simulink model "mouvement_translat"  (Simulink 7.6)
settings: Solver=ode15s  StartTime=0.0  StopTime=5  RelTol=1e-3
StopFcn:
  | close all
  | load pos_vit.mat
  | plot(pv(1,:),pv(2,:))
  | hold on
  | plot(pv(1,:),pv(3,:))
  | 
  | title('Position et vitesse')
  | grid
libraries: fl_lib x8, nesl_utility x5, elec_lib x1

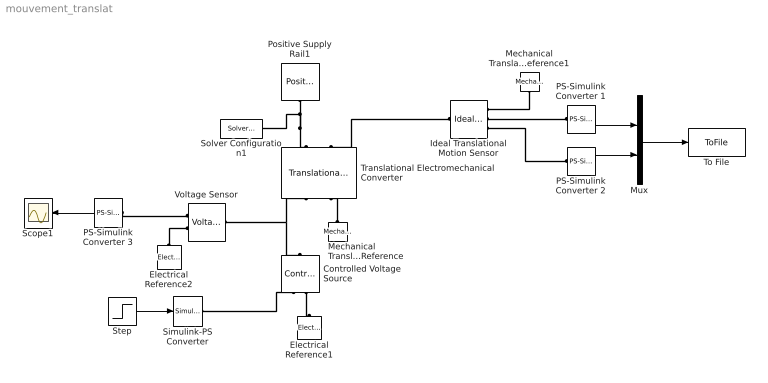
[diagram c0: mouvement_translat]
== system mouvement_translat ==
  Controlled Voltage Source : fl_lib/Electrical/Electrical Sources/Controlled Voltage Source  DialogController=NetworkEngine.DynNeDlgSource  SystemSampleTime=-1  i_Log=off  v_Log=off  LocalVarNames=|i|v  LocalVarDescs=|i|v  LocalVarLogging=[0 0]
  Electrical Reference1 : fl_lib/Electrical/Electrical Elements/Electrical Reference  DialogController=NetworkEngine.DynNeDlgSource  SystemSampleTime=-1  i_Log=off  LocalVarNames=|i  LocalVarDescs=|i  LocalVarLogging=[]
  Electrical Reference2 : fl_lib/Electrical/Electrical Elements/Electrical Reference  DialogController=NetworkEngine.DynNeDlgSource  SystemSampleTime=-1  i_Log=off  LocalVarNames=|i  LocalVarDescs=|i  LocalVarLogging=[]
  Ideal Translational Motion Sensor : fl_lib/Mechanical/Mechanical Sensors/Ideal Translational Motion Sensor  DialogController=NetworkEngine.DynNeDlgSource  SystemSampleTime=-1  offset=0 m  v_Log=off  f_Log=off  x_Log=off  LocalVarNames=|v|f|x  LocalVarDescs=|v|f|x  LocalVarLogging=[0 0 0]
  Mechanical Translational Reference : fl_lib/Mechanical/Translational Elements/Mechanical Translational Reference  DialogController=NetworkEngine.DynNeDlgSource  SystemSampleTime=-1  f_Log=off  LocalVarNames=|f  LocalVarDescs=|f  LocalVarLogging=0
  Mechanical Translational Reference1 : fl_lib/Mechanical/Translational Elements/Mechanical Translational Reference  DialogController=NetworkEngine.DynNeDlgSource  SystemSampleTime=-1  f_Log=off  LocalVarNames=|f  LocalVarDescs=|f  LocalVarLogging=0
  Mux : Mux  Inputs=2
  PS-Simulink Converter 1 : nesl_utility/PS-Simulink Converter  DialogController=NetworkEngine.DynNeUtilDlgSource  SystemSampleTime=-1  PhysicalDomain=network_engine_domain  LeftPortType=input  RightPortType=output  SubClassName=ps_output  Unit=m/s  AffineConversion=off
  PS-Simulink Converter 2 : nesl_utility/PS-Simulink Converter  DialogController=NetworkEngine.DynNeUtilDlgSource  SystemSampleTime=-1  PhysicalDomain=network_engine_domain  LeftPortType=input  RightPortType=output  SubClassName=ps_output  Unit=m  AffineConversion=off
  PS-Simulink Converter 3 : nesl_utility/PS-Simulink Converter  DialogController=NetworkEngine.DynNeUtilDlgSource  SystemSampleTime=-1  PhysicalDomain=network_engine_domain  LeftPortType=input  RightPortType=output  SubClassName=ps_output  Unit=V  AffineConversion=off
  Positive Supply Rail1 : elec_lib/Sources/Positive Supply Rail  DialogController=NetworkEngine.DynNeDlgSource  SystemSampleTime=-1  v0=12 V  current_Log=off  voltage_Log=off  power_Log=off  LocalVarNames=|current|voltage|power  LocalVarDescs=|Current (A)|Voltage (V)|Power (W)  LocalVarLogging=[0 0 0]
  Scope1 : Scope
  Simulink-PS Converter : nesl_utility/Simulink-PS Converter  DialogController=NetworkEngine.DynNeUtilDlgSource  SystemSampleTime=-1  PhysicalDomain=network_engine_domain  LeftPortType=input  RightPortType=output  SubClassName=ps_input  Unit=1  AffineConversion=off  InputFilterTimeConstant=.001  UdotUserProvided=0
  Solver Configuration1 : nesl_utility/Solver Configuration  DialogController=NetworkEngine.DynNeUtilDlgSource  SystemSampleTime=-1  PhysicalDomain=network_engine_domain  LeftPortType=input  RightPortType=generic  SubClassName=solver  Accelerate=off  Profile=off  ResidualTolerance=1e-9  MaxNonlinIter=12  MaxModeIter=2  DoFixedCost=off  UseLocalSampling=off  DoDC=off  LinearAlgebra=Sparse  LocalSolverSampleTime=.001  LocalSolverChoice=NE_BACKWARD_EULER_ADVANCER  UseLocalSolver=off
  Step : Step  Time=0.5  Before=12  After=0  SampleTime=0
  To File : ToFile  Filename=pos_vit.mat  MatrixName=pv
  Translational Electromechanical Converter : fl_lib/Electrical/Electrical Elements/Translational Electromechanical Converter  DialogController=NetworkEngine.DynNeDlgSource  SystemSampleTime=-1  K=0.1 s*V/m  i_Log=off  v_Log=off  f_Log=off  u_Log=off  LocalVarNames=|i|v|f|u  LocalVarDescs=|i|v|f|u  LocalVarLogging=[0 0 0 0]
  Voltage Sensor : fl_lib/Electrical/Electrical Sensors/Voltage Sensor  DialogController=NetworkEngine.DynNeDlgSource  SystemSampleTime=-1  i1_Log=off  v1_Log=off  LocalVarNames=|i1|v1  LocalVarDescs=|i1|v1  LocalVarLogging=[0 0]
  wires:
  PS-Simulink Converter 1/1 -> Mux/1
  PS-Simulink Converter 2/1 -> Mux/2
  Mux/1 -> To File/1
  Step/1 -> Simulink-PS Converter/1
  PS-Simulink Converter 3/1 -> Scope1/1
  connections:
  Voltage Sensor/LConn1 -- Translational Electromechanical Converter/RConn1 -- Controlled Voltage Source/LConn1
  Positive Supply Rail1/RConn1 -- Translational Electromechanical Converter/LConn1 -- Solver Configuration1/RConn1
  Ideal Translational Motion Sensor/LConn1 -- Translational Electromechanical Converter/LConn2
  Mechanical Translational Reference/LConn1 -- Translational Electromechanical Converter/RConn2
  Mechanical Translational Reference1/LConn1 -- Ideal Translational Motion Sensor/RConn1
  Ideal Translational Motion Sensor/RConn2 -- PS-Simulink Converter 1/LConn1
  Ideal Translational Motion Sensor/RConn3 -- PS-Simulink Converter 2/LConn1
  Electrical Reference2/LConn1 -- Voltage Sensor/RConn2
  PS-Simulink Converter 3/LConn1 -- Voltage Sensor/RConn1
  Controlled Voltage Source/RConn2 -- Electrical Reference1/LConn1
  Simulink-PS Converter/RConn1 -- Controlled Voltage Source/RConn1
